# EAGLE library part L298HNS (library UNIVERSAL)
L298HNS Puzdro pre povrchovu montaz,original usporiadanie pinov.
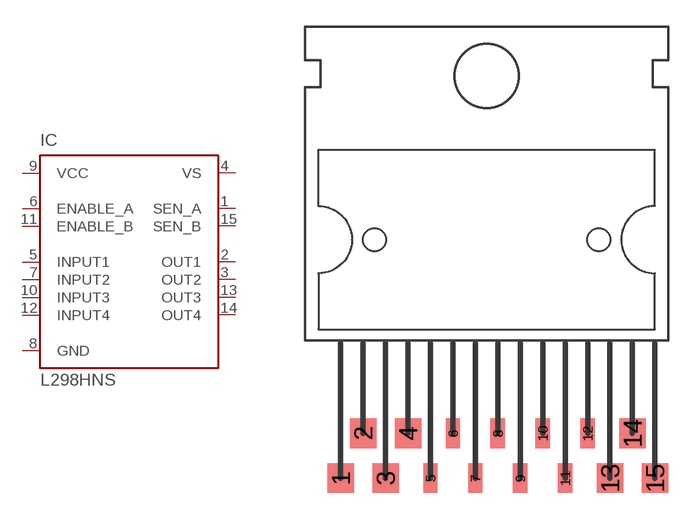
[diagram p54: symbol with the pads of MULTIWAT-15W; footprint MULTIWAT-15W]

Designator prefix IC

## L298HNS  [MULTIWAT-15W]
1  SEN_A  in
2  OUT1  out
3  OUT2  out
4  VS  pwr
5  INPUT1  in
6  ENABLE_A  in
7  INPUT2  in
8  GND  pwr
9  VCC  pwr
10  INPUT3  in
11  ENABLE_B  in
12  INPUT4  in
13  OUT3  out
14  OUT4  out
15  SEN_B  in

## Footprint MULTIWAT-15W (pad centres in mm)
smd 1.5 x 1.676: 1 1.27,-7.62; 2 2.54,-5.08; 3 3.81,-7.62; 4 5.08,-5.08; 13 16.51,-7.62; 14 17.78,-5.08; 15 19.05,-7.62
smd 0.813 x 1.676: 5 6.35,-7.62; 6 7.62,-5.08; 7 8.89,-7.62; 8 10.16,-5.08; 9 11.43,-7.62; 10 12.7,-5.08; 11 13.97,-7.62; 12 15.24,-5.08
